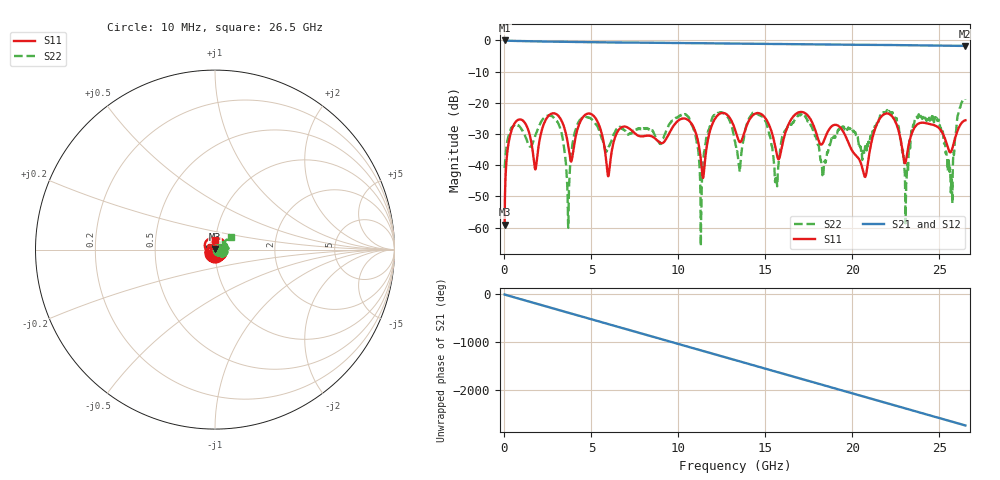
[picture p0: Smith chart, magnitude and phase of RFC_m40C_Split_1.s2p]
!Keysight Technologies,N5245B,MY55451909,A.13.80.08
!Automatic Fixture Removal (AFR)
!Date: Thursday, August 27, 2020, 03:54:04
!S2P File: Measurements: S11,S21,S12,S22:
# MHz S  RI  R 50
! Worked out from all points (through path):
!   2650 points, 10 MHz to 26.5 GHz, reference 50 ohm
!   highest |S21| = 0.00 dB at 10 MHz (marker M1); lowest = -1.7 dB at 26.47 GHz (marker M2)
!   group delay of S21, straight-line fit = 286 ps
!   lowest |S11| = -59.0 dB at 10 MHz (marker M3), VSWR 1.00, Z = 50 + j0.112 ohm
!   |S11| at or under -10 dB: start of sweep to end of sweep
!   |S22| runs from -65.9 to -18.8 dB; largest |S21 - S12| = 1.4e-15
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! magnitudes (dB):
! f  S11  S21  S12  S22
! 10 MHz  -59.0  0.0  0.0  -40.8
! 680 MHz  -25.9  -0.2  -0.2  -27.0
! 1.78 GHz  -41.3  -0.3  -0.3  -30.4
! 2.94 GHz  -23.5  -0.4  -0.4  -25.3
! 3.66 GHz  -33.5  -0.4  -0.4  -59.1
! 4.43 GHz  -25.3  -0.5  -0.5  -25.0
! 5.97 GHz  -43.5  -0.6  -0.6  -34.4
! 8.84 GHz  -32.3  -0.8  -0.8  -32.3
! 10.5 GHz  -25.3  -0.9  -0.9  -24.2
! 11.32 GHz  -39.7  -0.9  -0.9  -55.2
! 12.03 GHz  -25.8  -0.9  -0.9  -24.0
! 13.26 GHz  -28.6  -1.0  -1.0  -32.6
! 14.79 GHz  -23.7  -1.1  -1.1  -24.2
! 15.63 GHz  -35.7  -1.1  -1.1  -45.5
! 17.67 GHz  -26.0  -1.2  -1.2  -27.8
! 20.72 GHz  -43.7  -1.4  -1.4  -34.7
! 22.09 GHz  -23.5  -1.5  -1.5  -22.8
! 23.08 GHz  -38.6  -1.5  -1.5  -50.7
! 23.83 GHz  -26.6  -1.6  -1.6  -23.8
! 25.66 GHz  -35.8  -1.7  -1.7  -48.7
! 26.47 GHz  -25.6  -1.7  -1.7  -18.8
! 26.5 GHz  -25.6  -1.7  -1.7  -19.0
